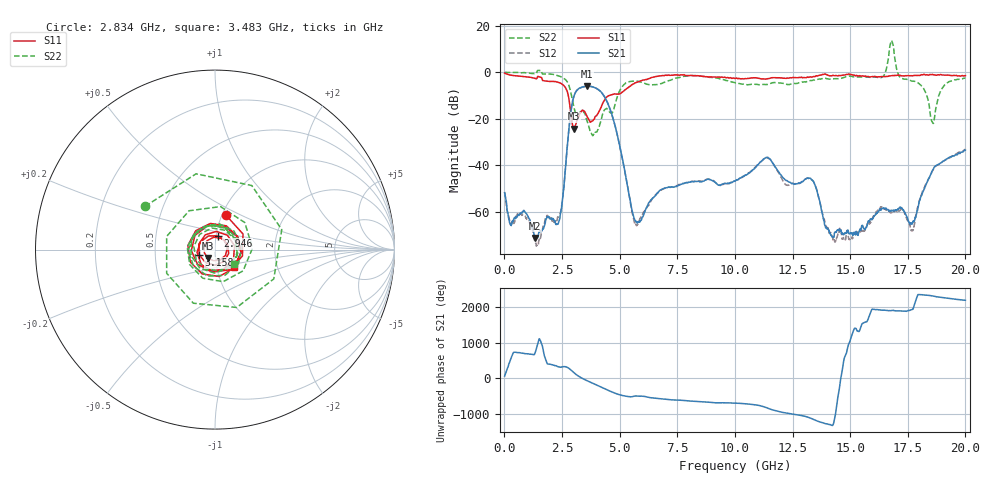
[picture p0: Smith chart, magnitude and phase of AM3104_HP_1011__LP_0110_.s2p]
!Created with skrf (http://scikit-rf.org).
# Hz S RI R 50.0
!freq ReS11 ImS11 ReS21 ImS21 ReS12 ImS12 ReS22 ImS22
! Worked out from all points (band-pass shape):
!   1601 points, 10 MHz to 20 GHz, reference 50 ohm
!   highest |S21| = -5.97 dB at 3.571 GHz (marker M1); lowest = -71.1 dB at 1.334 GHz (marker M2)
!   |S21| within 3 dB of the highest: 3.07 GHz to 4.235 GHz (1.166 GHz wide, 31.9 % of centre)
!   lowest |S11| = -24.2 dB at 3.021 GHz (marker M3), VSWR 1.13, Z = 46 - j4.36 ohm
!   |S11| at or under -10 dB: 2.773 GHz to 4.544 GHz (1.771 GHz wide, 48.4 % of centre)
!   |S22| runs from -27.3 to 13.6 dB; largest |S21 - S12| = 0.029
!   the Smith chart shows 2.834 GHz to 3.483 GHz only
!   S11 on the Smith chart (normalised r, x): 2.834 GHz: 1.04, +0.42; 2.946 GHz: 1.02, +0.16; 3.158 GHz: 0.84, -0.05; 3.483 GHz: 1.21, -0.24
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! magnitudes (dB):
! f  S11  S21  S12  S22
! 10 MHz  -0.4  -51.7  -51.6  0.0
! 1.334 GHz  -2.6  -71.1  -73.2  -0.6
! 2.371 GHz  -4.4  -63.8  -61.5  -1.6
! 2.834 GHz  -13.9  -21.1  -21.1  -6.8
! 2.946 GHz  -22.1  -13.2  -13.2  -11.7
! 3.021 GHz  -24.2  -10.2  -10.2  -15.2
! 3.158 GHz  -20.7  -7.6  -7.7  -18.5
! 3.346 GHz  -16.7  -6.5  -6.5  -16.4
! 3.483 GHz  -16.9  -6.1  -6.2  -17.6
! 3.571 GHz  -18.7  -6.0  -6.1  -20.3
! 4.57 GHz  -9.9  -15.4  -15.6  -17.2
! 5.695 GHz  -4.5  -64.2  -65.0  -3.7
! 6.682 GHz  -1.6  -51.4  -51.5  -5.2
! 10.01 GHz  -2.7  -46.7  -46.7  -4.5
! 11.39 GHz  -2.9  -36.6  -36.8  -5.3
! 13.34 GHz  -2.1  -46.3  -46.2  -3.6
! 14.32 GHz  -1.5  -69.0  -71.6  -2.8
! 16.68 GHz  -1.6  -59.5  -59.7  7.2
! 17.71 GHz  -1.5  -64.5  -68.0  -3.8
! 18.58 GHz  -1.0  -42.1  -42.3  -21.6
! 19.05 GHz  -1.2  -38.1  -38.1  -6.1
! 20 GHz  -1.5  -33.5  -33.1  -2.5
